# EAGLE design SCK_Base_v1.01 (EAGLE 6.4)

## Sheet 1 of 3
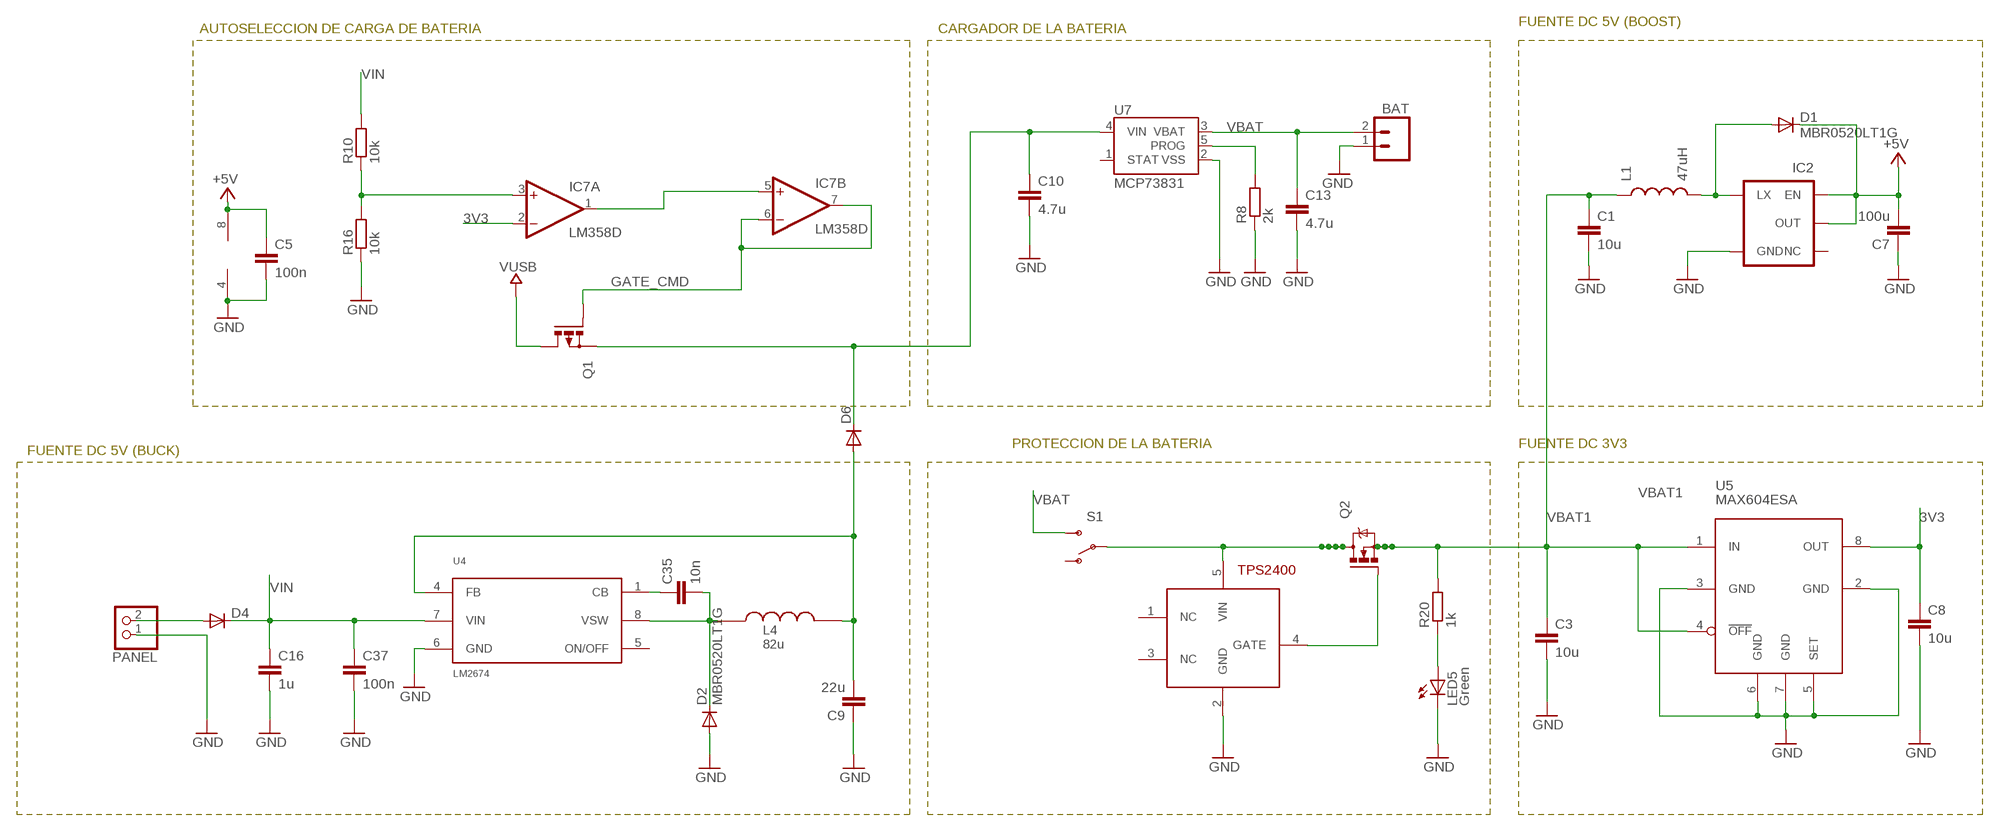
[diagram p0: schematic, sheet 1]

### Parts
BAT  M02-JST-2MM-SMT  [S2B-PH]
C1  10u  C-EUC0805  [C0805]
C3  10u  C-EUC0805  [C0805]
C5  100n  C-EUC0805  [C0805]
C7  100u  C-EUC1206  [C1206]
C8  10u  C-EUC0805  [C0805]
C9  22u  C-EUC1206  [C1206]
C10  4.7u  C-EUC0805  [C0805]
C13  4.7u  C-EUC0805  [C0805]
C16  1u  C-EUC0805  [C0805]
C35  10n  C-EUC0805  [C0805]
C37  100n  C-EUC0805  [C0805]
D1  MBR0520LT1G  DIODE-SOD123  [SOD123]
D2  MBR0520LT1G  DIODE-SOD123  [SOD123]
D4  DIODESMA-ALT  [SMA-DIODE_ALT]
D6  DIODESMA-ALT  [SMA-DIODE_ALT]
IC2  V_REG_NCP1400SOT23-5  [SOT23-5]
IC7  LM358D  [SO08]
L1  47uH  INDUCTORCR54  [CR54]
L4  82u  LSDR1006  [SDR1006]
LED5  Green  LEDCHIP-LED0805  [CHIP-LED0805]
PANEL  PINHD-1X2  [1X02]
Q1  P-MOSFET-SO8  [SO-08]
Q2  N-MOSFET-SO8S  [SO-08]
R8  2k  R-EU_R0805  [R0805]
R10  10k  R-EU_R0805  [R0805]
R16  10k  R-EU_R0805  [R0805]
R20  1k  R-EU_R0805  [R0805]
S1  SWITCH-SPST-SMD-A  [SWITCH-SPST-SMD-A]
U3  TPS2400  [SOT23-5L]
U4  LM2674  [SO8]
U5  MAX604ESA  [SO-08]
U7  MCP73831  [SOT23-5]

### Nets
3V3: C8.1 IC7.2(A:-IN) U5.8(OUT) ; also sheet 3
+5V [usbvcc]: C5.1 C7.2 D1.C IC2.1(EN) IC2.2(OUT) IC7.8(P:V+) ; also sheet 2,3
GATE_CMD: IC7.6(B:-IN) IC7.7(B:OUT) Q1.4(G)
GND: BAT.1 C1.2 C3.2 C5.2 C7.1 C8.2 C9.1 C10.2 C13.2 C16.2 C37.2 D2.A IC2.4(GND) IC7.4(P:V-) LED5.C PANEL.1 R8.1 R16.1 U3.2(GND) U4.6(GND) U5.2(GND) U5.3(GND) U5.5(SET) U5.6(GND) U5.7(GND) U7.2(VSS) ; also sheet 2,3
N$3 [power]: D4.A PANEL.2
N$5: IC7.3(A:+IN) R10.1 R16.2
N$7: IC7.1(A:OUT) IC7.5(B:+IN)
N$10 [usbvcc]: C9.2 D6.A L4.2 U4.4(FB)
N$13: R8.2 U7.5(PROG)
N$19 [usbvcc]: C10.1 D6.C Q1.1(S) Q1.2(S) Q1.3(S) U7.4(VIN)
N$20: LED5.A R20.1
N$30: Q2.4(G) U3.4(GATE)
N$31: D1.A IC2.5(LX) L1.P$2
N$47: C35.1 U4.1(CB)
N$54: C35.2 D2.C L4.1 U4.8(VSW)
VBAT: BAT.2 C13.1 S1.3(S) U7.3(VBAT)
VBAT1: C1.1 C3.1 L1.P$1 Q2.1(S) Q2.2(S) Q2.3(S) R20.2 U5.1(IN) U5.4(!OFF) ; also sheet 2
VIN [power]: C16.1 C37.1 D4.C R10.2 U4.7(VIN) ; also sheet 3
VTPS: Q2.5(D) Q2.6(D) Q2.7(D) Q2.8(D) S1.2(P) U3.5(VIN)
VUSB: Q1.5(D) Q1.6(D) Q1.7(D) Q1.8(D) ; also sheet 2
Unconnected: IC2.3(NC) S1.1(O) U3.1(NC) U3.3(NC) U4.5(ON/OFF) U7.1(STAT)

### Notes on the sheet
- FUENTE DC 5V (BOOST)
- AUTOSELECCION DE CARGA DE BATERIA | CARGADOR DE LA BATERIA
- PROTECCION DE LA BATERIA | FUENTE DC 3V3
- FUENTE DC 5V (BUCK)

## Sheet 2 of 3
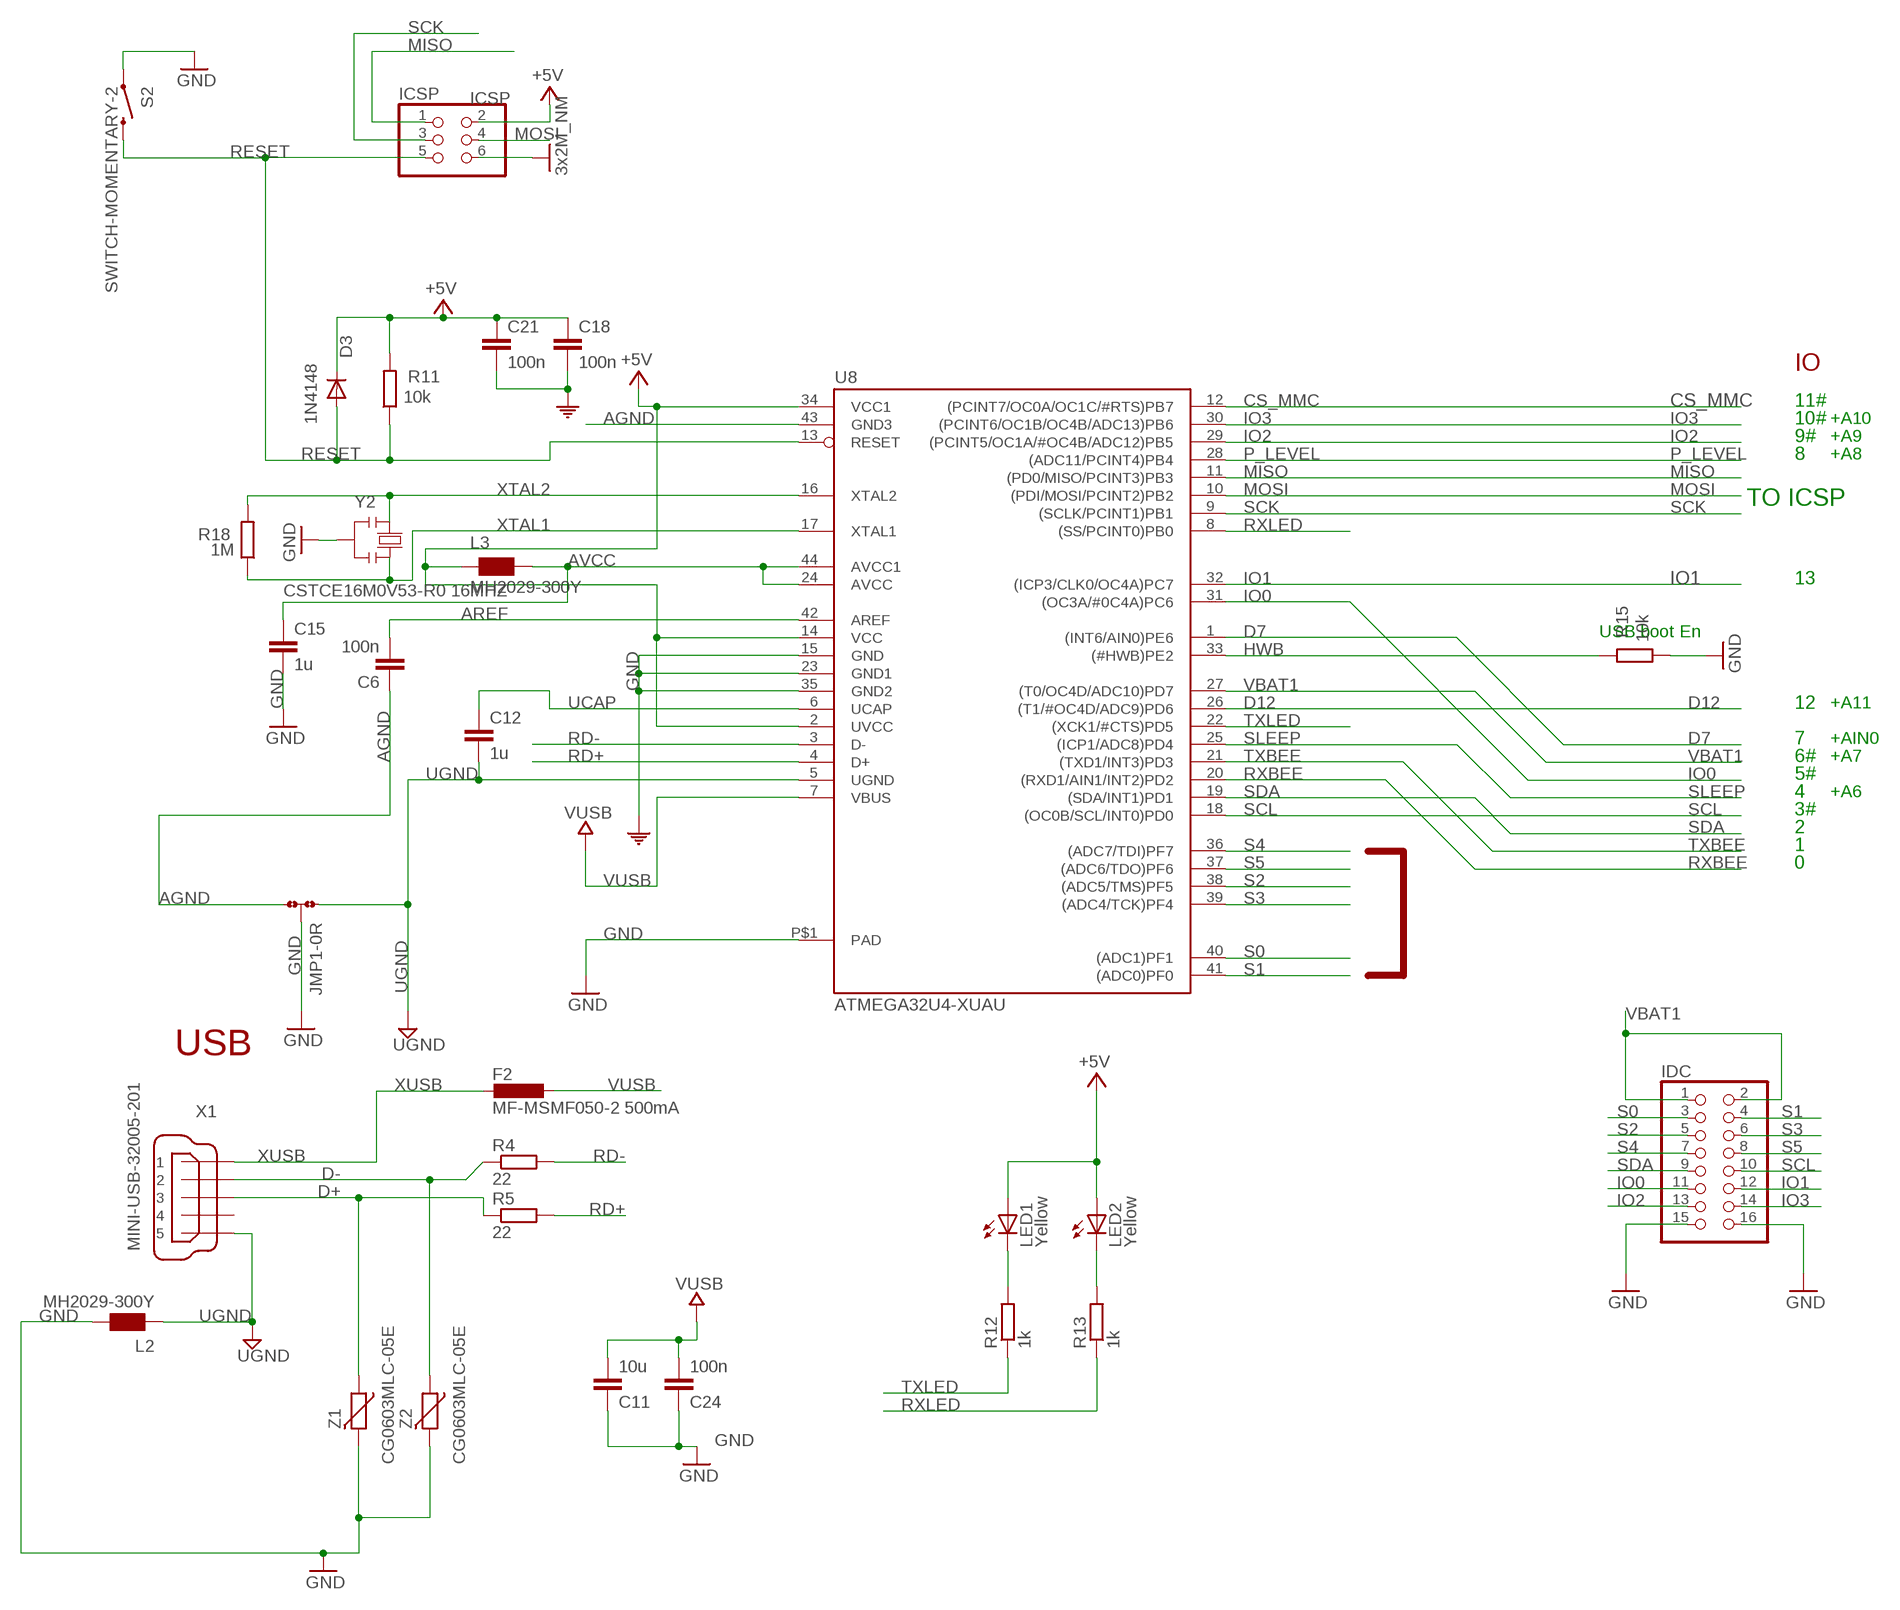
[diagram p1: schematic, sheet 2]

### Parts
C6  100n  C-EUC0805  [C0805]
C11  10u  C-EUC0805  [C0805]
C12  1u  C-EUC0805  [C0805]
C15  1u  C-EUC0805  [C0805]
C18  100n  C-EUC0805  [C0805]
C21  100n  C-EUC0805  [C0805]
C24  100n  C-EUC0805  [C0805]
D3  1N4148  DIODE-SOD123  [SOD123]
F2  MF-MSMF050-2 500mA  L-EUL1812  [L1812]
ICSP  ICSP  PINHD-2X3  [2X03]
IDC  PINHD-2X8  [2X08]
JMP1  0R-JUMPC  [C0R-JMP]
L2  MH2029-300Y  WE-CBF_0805  [0805]
L3  MH2029-300Y  WE-CBF_0805  [0805]
LED1  Yellow  LEDCHIP-LED0805  [CHIP-LED0805]
LED2  Yellow  LEDCHIP-LED0805  [CHIP-LED0805]
R4  22  R-EU_R0805  [R0805]
R5  22  R-EU_R0805  [R0805]
R11  10k  R-EU_R0805  [R0805]
R12  1k  R-EU_R0805  [R0805]
R13  1k  R-EU_R0805  [R0805]
R15  10k  R-EU_R0805  [R0805]
R18  1M  R-EU_R0805  [R0805]
S2  SWITCH-MOMENTARY-2  [TACTILE_SWITCH_TALL]
U8  ATMEGA32U4-XUAU  [TQFP44-PAD]
X1  MINI-USB-32005-201  [32005-201]
Y2  CSTCE16M0V53-R0 16MHZ  RESONATORMU  [RESONATOR]
Z1  CG0603MLC-05E  VARISTORCN0603  [CT/CN0603]
Z2  CG0603MLC-05E  VARISTORCN0603  [CT/CN0603]

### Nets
+5V [usbvcc]: C18.1 C21.1 D3.C ICSP.2 L3.1 LED1.A LED2.A R11.2 U8.2(UVCC) U8.14(VCC) U8.34(VCC1) ; also sheet 1,3
AGND: C6.1 JMP1.3 U8.43(GND3)
AREF [aref]: C6.2 U8.42(AREF)
AVCC: C15.1 L3.2 U8.24(AVCC) U8.44(AVCC1)
CS_MMC: U8.12((PCINT7/OC0A/OC1C/#RTS)PB7) ; also sheet 3
D7: U8.1((INT6/AIN0)PE6)
D12: U8.26((T1/#OC4D/ADC9)PD6)
D+: R5.1 X1.3 Z1.1
D-: R4.1 X1.2 Z2.1
GND: C11.1 C15.2 C18.2 C21.2 C24.1 ICSP.6 IDC.15 IDC.16 JMP1.2 L2.2 R15.1 S2.A2 U8.15(GND) U8.23(GND1) U8.35(GND2) U8.P$1(PAD) Y2.2 Z1.2 Z2.2 ; supply symbol labelled 3x2M_NM, COM ; also sheet 1,3
HWB: R15.2 U8.33((#HWB)PE2)
IO0: IDC.11 U8.31((OC3A/#0C4A)PC6)
IO1: IDC.12 U8.32((ICP3/CLK0/OC4A)PC7)
IO2: IDC.13 U8.29((PCINT5/OC1A/#OC4B/ADC12)PB5)
IO3: IDC.14 U8.30((PCINT6/OC1B/OC4B/ADC13)PB6)
MISO: ICSP.1 U8.11((PD0/MISO/PCINT3)PB3) ; also sheet 3
MOSI: ICSP.4 U8.10((PDI/MOSI/PCINT2)PB2) ; also sheet 3
N$2 [usbvcc]: LED1.C R12.2
N$4 [usbvcc]: LED2.C R13.2
P_LEVEL: U8.28((ADC11/PCINT4)PB4) ; also sheet 3
RD+: R5.2 U8.4(D+)
RD-: R4.2 U8.3(D-)
RESET: D3.A ICSP.5 R11.1 S2.B2 U8.13(RESET) ; also sheet 3
RXBEE: U8.20((RXD1/AIN1/INT2)PD2) ; also sheet 3
RXLED: R13.1 U8.8((SS/PCINT0)PB0)
S0: IDC.3 U8.40((ADC1)PF1)
S1: IDC.4 U8.41((ADC0)PF0)
S2: IDC.5 U8.38((ADC5/TMS)PF5)
S3: IDC.6 U8.39((ADC4/TCK)PF4)
S4: IDC.7 U8.36((ADC7/TDI)PF7)
S5: IDC.8 U8.37((ADC6/TDO)PF6)
SCK: ICSP.3 U8.9((SCLK/PCINT1)PB1) ; also sheet 3
SCL: IDC.10 U8.18((OC0B/SCL/INT0)PD0) ; also sheet 3
SDA: IDC.9 U8.19((SDA/INT1)PD1) ; also sheet 3
SLEEP: U8.25((ICP1/ADC8)PD4) ; also sheet 3
TXBEE: U8.21((TXD1/INT3)PD3) ; also sheet 3
TXLED: R12.1 U8.22((XCK1/#CTS)PD5)
UCAP: C12.1 U8.6(UCAP)
UGND [gnd]: C12.2 JMP1.1 L2.1 U8.5(UGND) X1.5
VBAT1: IDC.1 IDC.2 U8.27((T0/OC4D/ADC10)PD7) ; also sheet 1
VUSB: C11.2 C24.2 F2.1 U8.7(VBUS) ; also sheet 1
XTAL1: R18.1 U8.17(XTAL1) Y2.3
XTAL2: R18.2 U8.16(XTAL2) Y2.1
XUSB [usbvcc]: F2.2 X1.1
Unconnected: X1.4

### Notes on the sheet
- IO
- 11#
- 10# | +A10
- 9# | +A9
- 8 | +A8
- TO ICSP
- 13
- USB boot En
- 12 | +A11
- 7 | +AIN0
- 6# | +A7
- 5#
- 4 | +A6
- 3#
- 2
- 1
- 0
- USB

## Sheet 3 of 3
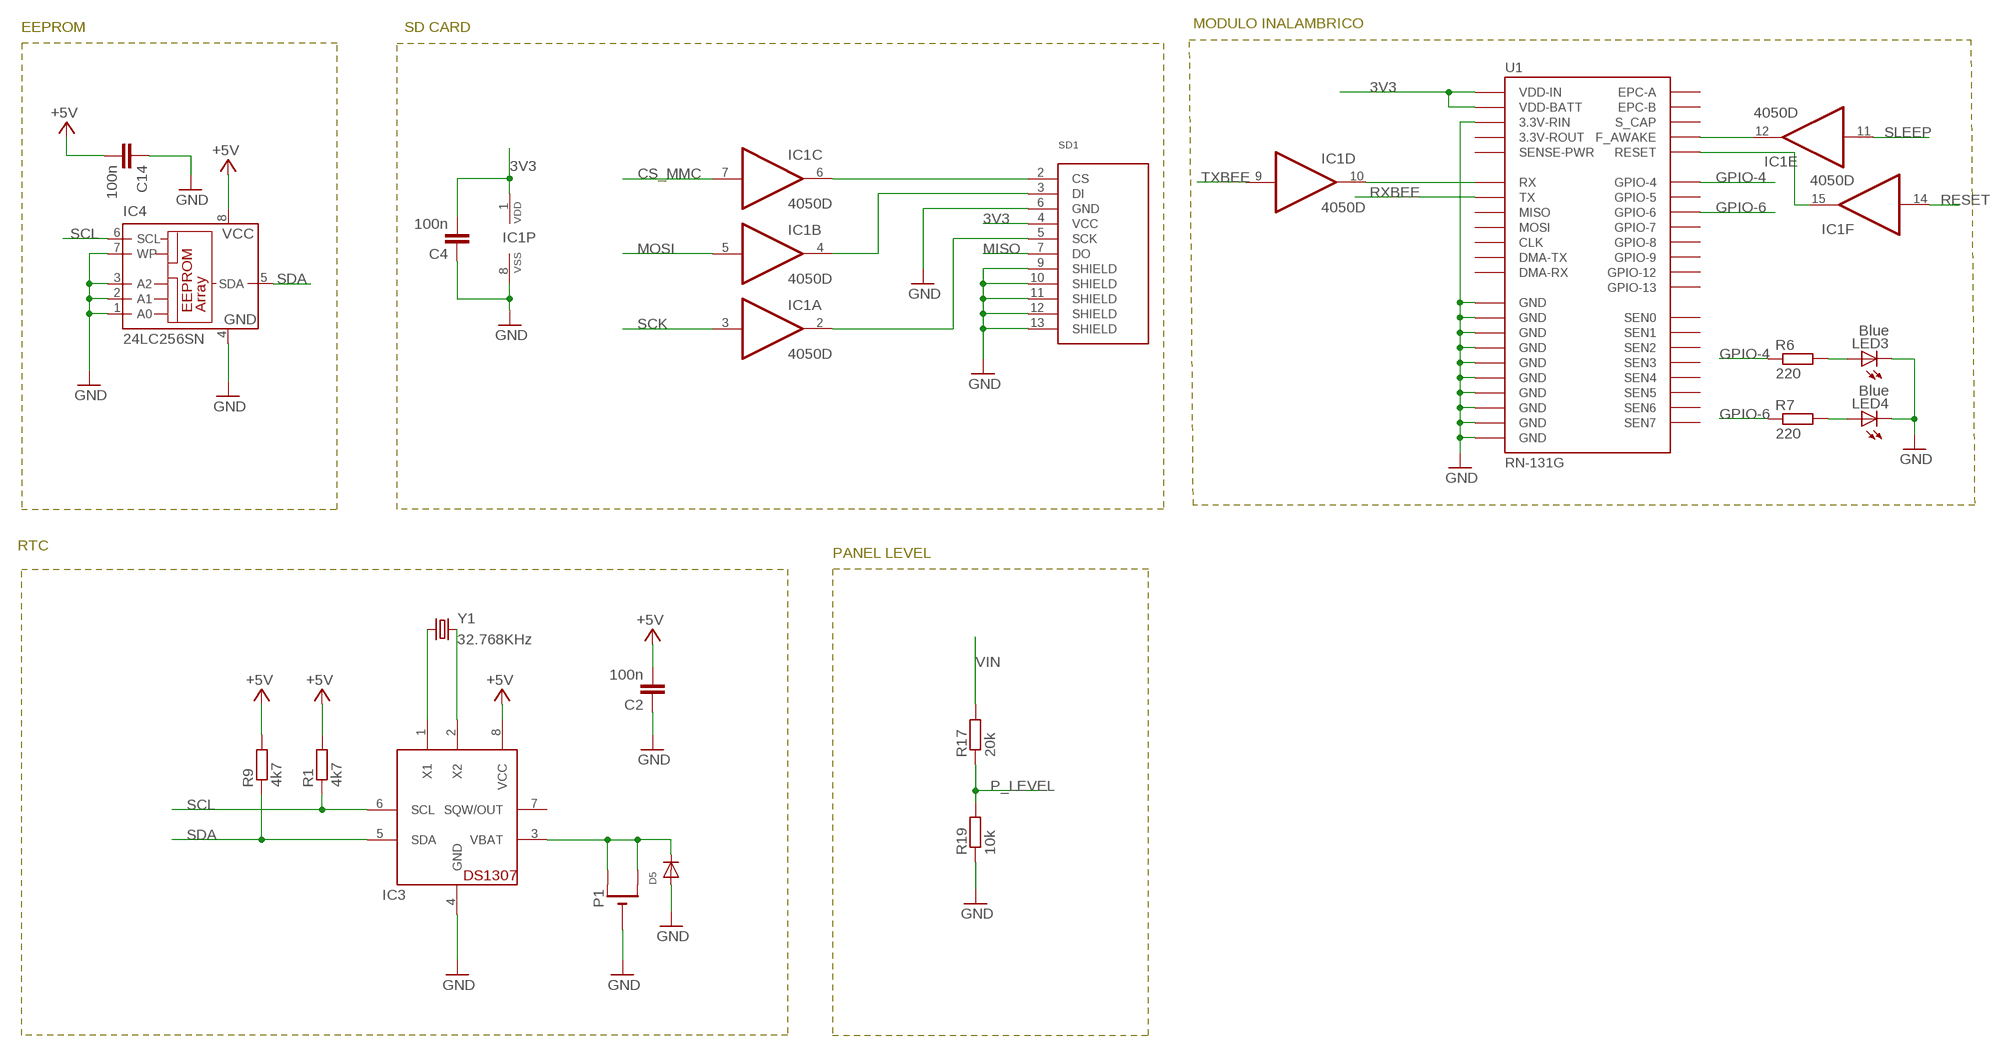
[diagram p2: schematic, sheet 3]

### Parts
C2  100n  C-EUC0805  [C0805]
C4  100n  C-EUC0805  [C0805]
C14  100n  C-EUC0805  [C0805]
D5  DIODESOD-323F  [SOD-323F]
IC1  4050D  [SO16]
IC3  DS1307SOIC  [SO08-SKINNYPADS]
IC4  24LC256SN  [SO-08]
LED3  Blue  LEDCHIP-LED0805  [CHIP-LED0805]
LED4  Blue  LEDCHIP-LED0805  [CHIP-LED0805]
P1  CR1220SMT  [CR1220-SMD]
R1  4k7  R-EU_R0805  [R0805]
R6  220  R-EU_R0805  [R0805]
R7  220  R-EU_R0805  [R0805]
R9  4k7  R-EU_R0805  [R0805]
R17  20k  R-EU_R0805  [R0805]
R19  10k  R-EU_R0805  [R0805]
SD1  SD_CARD_SOCKETDM3CS  [DM3CS]
U1  RN-131G  [RN-131G]
Y1  32.768KHz  CRYSTALABS10  [ABS10]

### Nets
3V3: C4.2 IC1.1(P:VDD) SD1.4(VCC) U1.P$20(VDD-BATT) U1.P$21(VDD-IN) ; also sheet 1
+5V [usbvcc]: C2.2 C14.2 IC3.8(VCC) IC4.8(VCC) R1.2 R9.2 ; also sheet 1,2
CS_MMC: IC1.7(C:I) ; also sheet 2
GND: C2.1 C4.1 C14.1 D5.A IC1.8(P:VSS) IC3.4(GND) IC4.1(A0) IC4.2(A1) IC4.3(A2) IC4.4(GND) IC4.7(WP) LED3.C LED4.C P1.- R19.1 SD1.6(GND) SD1.9(SHIELD) SD1.10(SHIELD) SD1.11(SHIELD) SD1.12(SHIELD) SD1.13(SHIELD) U1.P$18(3.3V-RIN) U1.P$19(GND) U1.P$36(GND) U1.P$37(GND) U1.P$38(GND) U1.P$39(GND) U1.P$40(GND) U1.P$41(GND) U1.P$42(GND) U1.P$43(GND) U1.P$44(GND) ; also sheet 1,2
GPIO-4: R6.1 U1.P$29(GPIO-4)
GPIO-6: R7.1 U1.P$27(GPIO-6)
MISO: SD1.7(DO) ; also sheet 2
MOSI: IC1.5(B:I) ; also sheet 2
N$1: IC1.10(D:O) U1.P$12(RX)
N$6: LED4.A R7.2
N$8: LED3.A R6.2
N$9: IC1.6(C:O) SD1.2(CS)
N$11: IC1.2(A:O) SD1.5(SCK)
N$12: IC1.4(B:O) SD1.3(DI)
N$14: IC1.12(E:O) U1.P$9(F_AWAKE)
N$15: IC1.15(F:O) U1.P$5(RESET)
N$16: IC3.1(X1) Y1.1
N$17: IC3.2(X2) Y1.2
N$18: D5.C IC3.3(VBAT) P1.+$1(+) P1.+$2(+1)
P_LEVEL: R17.1 R19.2 ; also sheet 2
RESET: IC1.14(F:I) ; also sheet 2
RXBEE: U1.P$13(TX) ; also sheet 2
SCK: IC1.3(A:I) ; also sheet 2
SCL: IC3.6(SCL) IC4.6(SCL) R1.1 ; also sheet 2
SDA: IC3.5(SDA) IC4.5(SDA) R9.1 ; also sheet 2
SLEEP: IC1.11(E:I) ; also sheet 2
TXBEE: IC1.9(D:I) ; also sheet 2
VIN [power]: R17.2 ; also sheet 1
Unconnected: IC3.7(SQW/OUT) U1.P$1(SEN6) U1.P$2(SEN4) U1.P$3(SEN5) U1.P$4(SEN7) U1.P$6(EPC-A) U1.P$7(EPC-B) U1.P$8(S_CAP) U1.P$10(GPIO-13) U1.P$11(GPIO-12) U1.P$14(MOSI) U1.P$15(CLK) U1.P$16(MISO) U1.P$17(3.3V-ROUT) U1.P$22(DMA-TX) U1.P$23(DMA-RX) U1.P$24(GPIO-9) U1.P$25(GPIO-8) U1.P$26(GPIO-7) U1.P$28(GPIO-5) U1.P$30(SEN1) U1.P$31(SEN2) U1.P$32(SEN3) U1.P$33(SENSE-PWR) U1.P$34(SEN0)

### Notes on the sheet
- EEPROM | SD CARD | MODULO INALAMBRICO
- RTC
- PANEL LEVEL

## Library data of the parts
BAT = SparkFun:M02: Header 2
C1-C5 C7-C10 C13 C14 C16 C35 C37 = rcl:C-EU: CAPACITOR, European symbol
C6 C11 C12 C15 C18 C21 C24 = SmartPrj:C-EU: CAPACITOR, European symbol
D1-D3 = diode:DIODE-: DIODE
D4 D6 = SparkFun-DiscreteSemi:DIODE: Diode
D5 = adafruit:DIODE: Diode
F2 = rcl:L-EU: INDUCTOR, European symbol
IC1 = 40xx:4050: Hex non-inverting BUFFER
IC2 = SparkFunEagle-3-30-09:V_REG_NCP1400: Switching step-up voltage regulator NCP1400 switiching regulator takes single cell AA and outputs 100mA at 3.3V or 5V with minimal number of external components.
IC3 = adafruit:DS1307: DS1307 Real time clock (RTC) with battery backup ability. Talk to it via i2c
IC4 = microchip:24*: Serial EEPROM I2C; MF: MICROCHIP; MPN: 24LC256-I/SN; OC_FARNELL: 9757996; OC_NEWARK: 27C9144
IC7 = linear:LM358: OP AMP also LM158; LM258; LM2904 Source: http://cache.national.com/ds/LM/LM158.pdf
ICSP = SmartPrj:PINHD-2X3: PIN HEADER
IDC = pinhead:PINHD-2X8: PIN HEADER
JMP1 = jump-0r-smd:0R-JUMP: SMD 0R 0805 Jumper
L1 = SparkFunEagle-3-30-09:INDUCTOR: Inductors
L2 L3 = wuerth-elektronik:WE-CBF: SMD EMI Suppression Ferrite Beads
L4 = Hangar:L
LED1-LED5 = led:LED: LED
P1 = adafruit:CR1220: CR1216/CR1220/CR1225 12mm 3V lithium coin cell Great for battery packup. Both SMT and THM holders. Note the THM package has the ground pads on both sides of the PCB so that the masks are the same - this reduces the cost
PANEL = pinhead:PINHD-1X2: PIN HEADER
Q1 = transistor-power:P-MOSFET-SO8: P-Channel MOSFET Example: FDS4435A; P-Channel Logic Level PowerTrench® MOSFET FDS4465; P-Channel 1.8V Specified PowerTrench® MOSFET Source: www.fairchildsemi.com
Q2 = transistor-power:N-MOSFET-SO8: N-Channel MOSFET Example: FDS7760A; N-Channel Logic Level PowerTrench® MOSFET FDS2572; N-Channel UltraFET® Trench MOSFET Source: www.fairchildsemi.com
R1 R4-R10 R12 R13 R16 R17 R19 R20 = rcl:R-EU_: RESISTOR, European symbol
R11 R15 R18 = SmartPrj:R-EU_: RESISTOR, European symbol
S1 = SparkFun 13-1-2012:SWITCH-SPST: SPST Switch Simple slide switch. Spark Fun Electronics SKU : COM-00102
S2 = SparkFun 13-1-2012:SWITCH-MOMENTARY-2
SD1 = Hangar:SD_CARD_SOCKET: SD/MMC Socket Media socket for SD and MMC cards. Push-push type. Model MOLEX 503182-0853
U1 = SparkFun:RN-131G: Roving Netowrks WiFLy GSX Module
U3 = texas-msp:TPS2400
U4 = Hangar:LM2674
U5 = Hangar:MAX604
U7 = SparkFun-PowerIC:MCP73831: Miniature single cell, fully integrated Li-Ion, Li-polymer charge management controller http://ww1.microchip.com/downloads/en/DeviceDoc/21984a.pdf
U8 = SmartPrj:ATMEGA32U4-XU
X1 = con-cypressindustries:MINI-USB-: MINI USB-B Conector Source: www.cypressindustries.com; OC_FARNELL: unknown; OC_NEWARK: unknown
Y1 = Hangar:CRYSTAL: CRYSTAL
Y2 = SmartPrj:RESONATOR
Z1 Z2 = varistor:VARISTOR: VARISTOR

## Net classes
1 power: width 0.254 mm, drill 0.6 mm, clearance 0.203 mm
2 gnd: width 0.254 mm, drill 0.6 mm, clearance 0.203 mm
3 usbvcc: width 0.254 mm, drill 0.6 mm, clearance 0.203 mm
4 aref: width 0.254 mm, drill 0.6 mm, clearance 0.203 mm

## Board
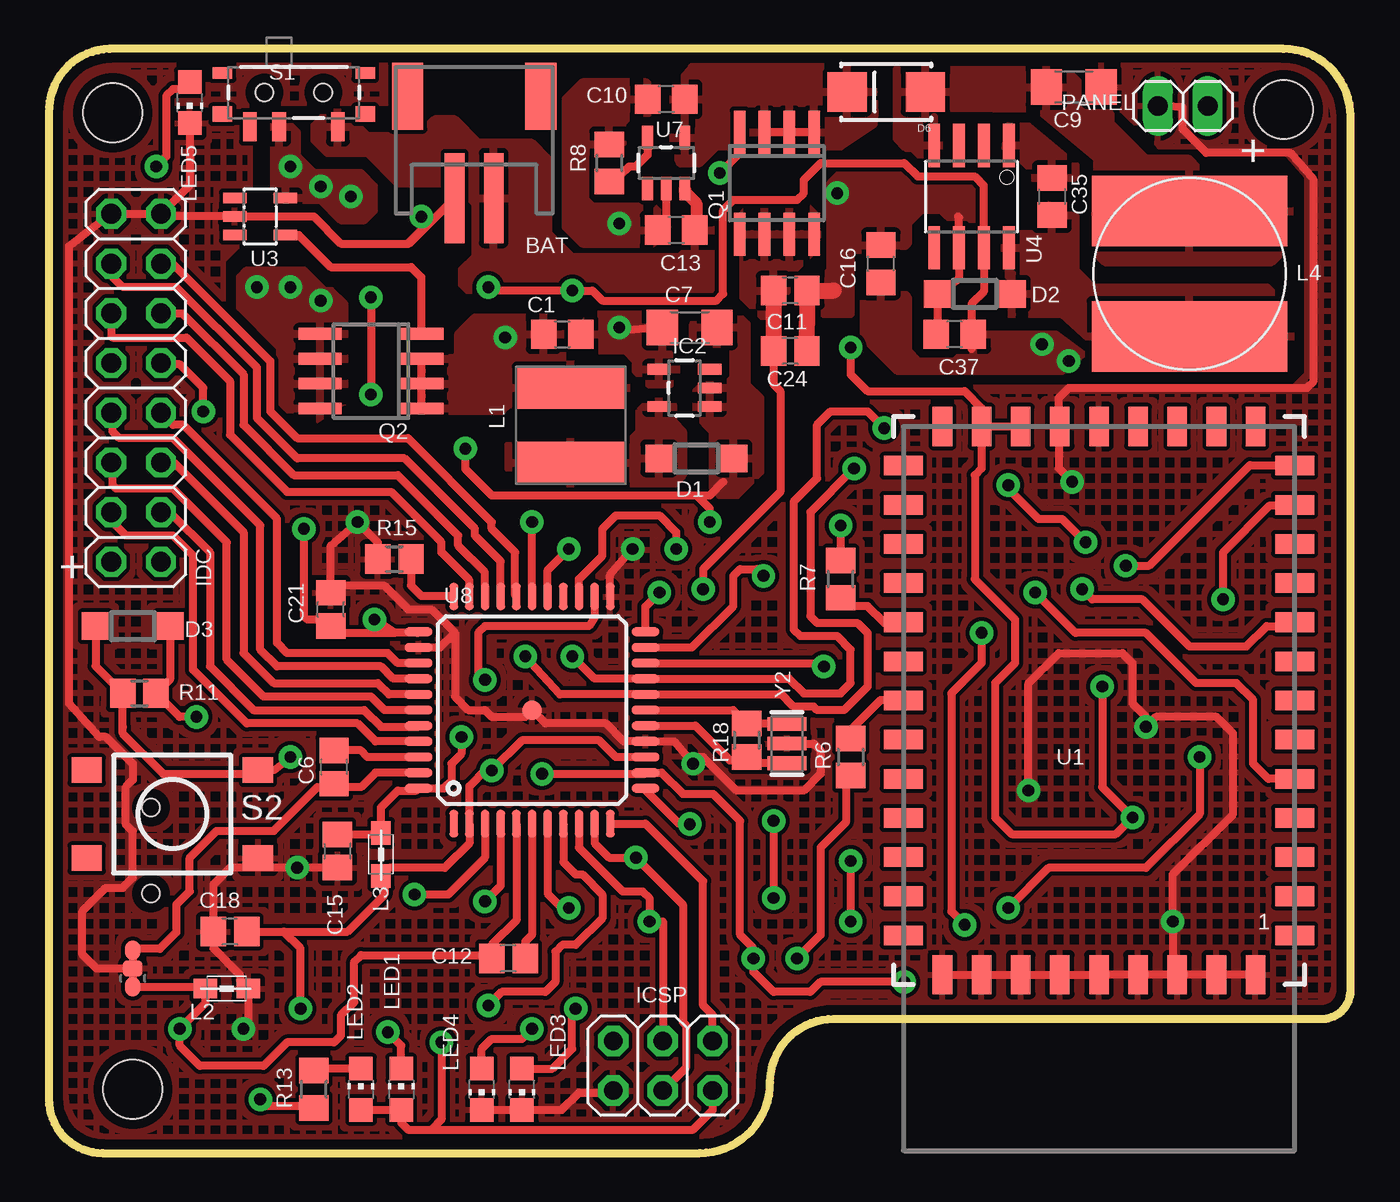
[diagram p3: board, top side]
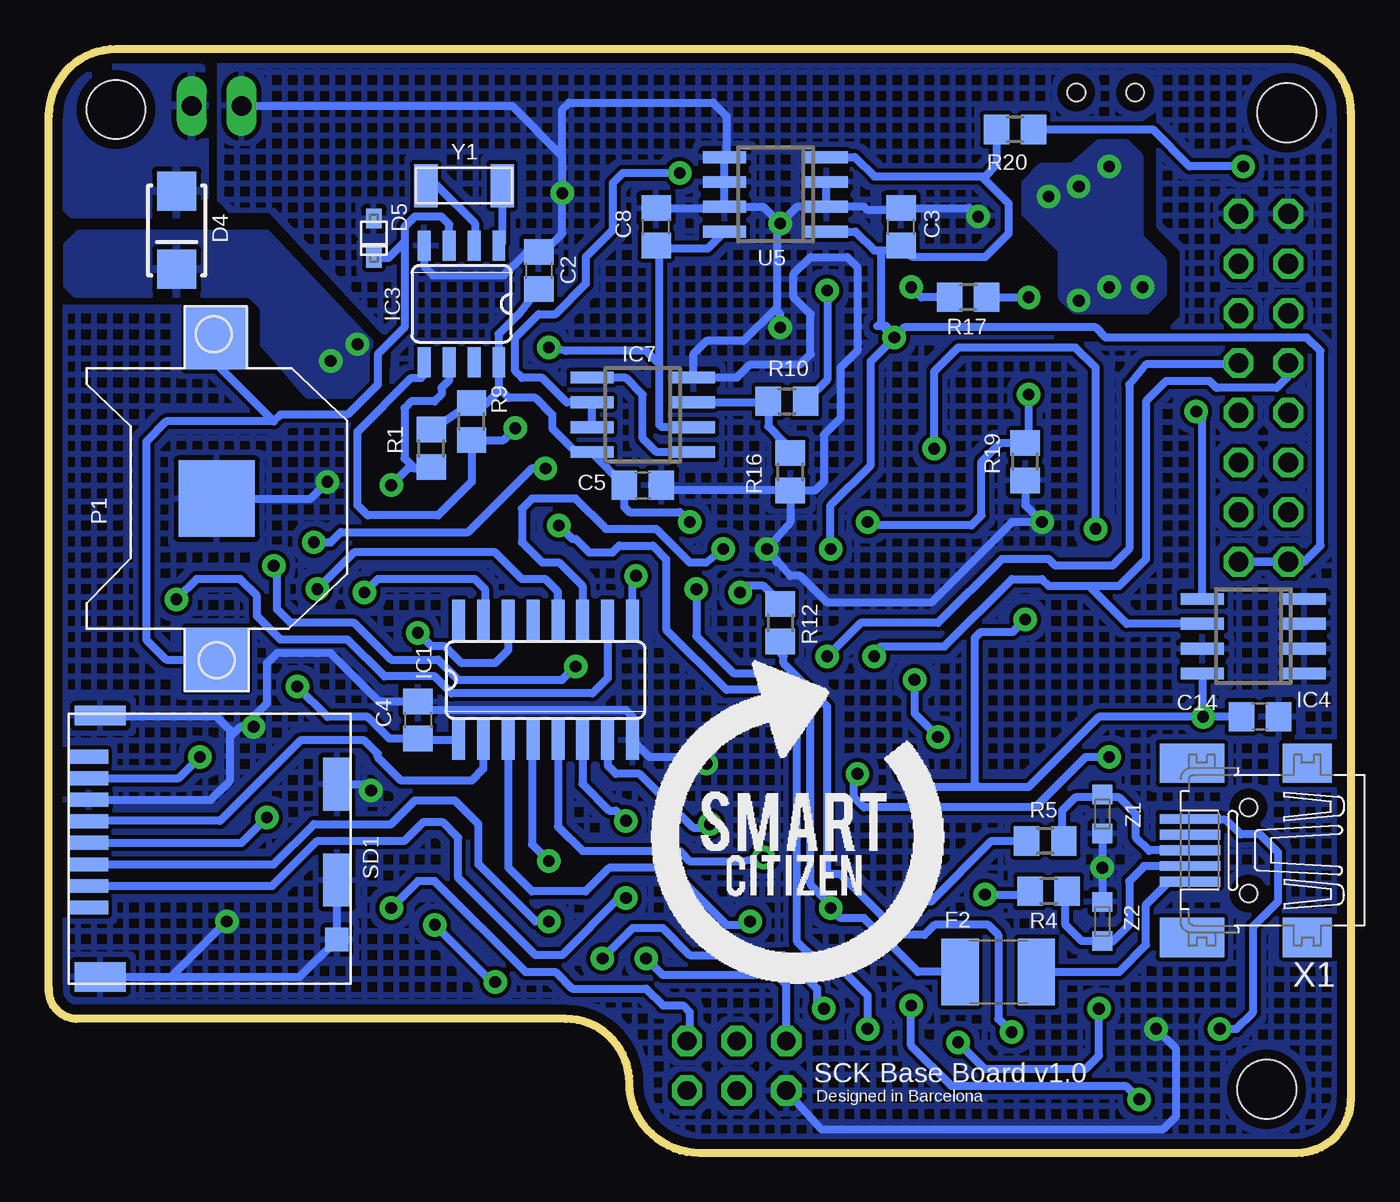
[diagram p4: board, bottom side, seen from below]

Size 66.52 x 56.41 mm. Coordinates in mm from the lower left corner, seen from the top.
Outline: 2.74,0 33.26,0 arc90 36.86,3.6 arc-90 40.12,6.86 65.15,6.86 arc90 66.52,8.4 66.52,52.98 arc90 63.09,56.41 3.09,56.41 arc90 0,53.15 0,2.74 arc90 2.74,0
Copper layers (1*16): Top 0.035mm / dielectric 1.5mm / Bottom 0.035mm
Design rules "default": minimum track width 6mil, minimum drill 0.6mm, track to track 8mil, track to pad 8mil, pad to pad 8mil, via to via 8mil, smd to smd 8mil, copper to edge 20mil, drill to drill 1mm, minimum pad ring 10mil, minimum via ring 0.3mm, stop-mask expansion 4mil, vias tented up to drill 0mil, thermal gap 10mil
Holes 3 mm at 3.26,53.15 4.29,3.26 63.09,53.32

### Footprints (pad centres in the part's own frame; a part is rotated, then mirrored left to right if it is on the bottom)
S2B-PH = smd 1 x 4.6: 1 -1,-3.7; 2 1,-3.7 | smd 1.6 x 3.4: NC1 -3.4,1.5; NC2 3.4,1.5
C0805 = smd 1.3 x 1.5: 1 -0.95,0; 2 0.95,0
C0805' = smd 1.3 x 1.5: 1 -0.85,0; 2 0.85,0
C1206 = smd 1.6 x 1.8: 1 -1.4,0; 2 1.4,0
SOD123 = smd 1.4 x 1.4: A 1.9,0; C -1.9,0
SMA-DIODE_ALT = smd 2 x 2: A -2,0; C 2,0
SOD-323F = smd 1 x 0.8: A -1,0; C 1,0
L1812 = smd 1.9 x 3.4: 1 -1.95,0; 2 1.95,0
SO16 = smd 0.66 x 2.032: 1 -4.445,-3.073; 2 -3.175,-3.073; 3 -1.905,-3.073; 4 -0.635,-3.073; 5 0.635,-3.073; 6 1.905,-3.073; 7 3.175,-3.073; 8 4.445,-3.073; 9 4.445,3.073; 10 3.175,3.073; 11 1.905,3.073; 12 0.635,3.073; 13 -0.635,3.073; 14 -1.905,3.073; 15 -3.175,3.073; 16 -4.445,3.073
SOT23-5 = smd 0.55 x 1.2: 1 -0.95,-1.3; 2 0,-1.3; 3 0.95,-1.3; 4 0.95,1.3; 5 -0.95,1.3
SO08-SKINNYPADS = smd 0.66 x 1.524: 1 -1.905,-2.973; 2 -0.635,-2.973; 3 0.635,-2.973; 4 1.905,-2.973; 5 1.905,2.973; 6 0.635,2.973; 7 -0.635,2.973; 8 -1.905,2.973
SO-08 = smd 0.6 x 2.2: 1 -1.905,-2.6; 2 -0.635,-2.6; 3 0.635,-2.6; 4 1.905,-2.6; 5 1.905,2.6; 6 0.635,2.6; 7 -0.635,2.6; 8 -1.905,2.6
SO08 = smd 0.6 x 2.2: 1 -1.905,-2.6; 2 -0.635,-2.6; 3 0.635,-2.6; 4 1.905,-2.6; 5 1.905,2.6; 6 0.635,2.6; 7 -0.635,2.6; 8 -1.905,2.6
2X03 = drill 0.95 pad 1.55 octagon: 1 -2.54,-1.27; 2 -2.54,1.27; 3 0,-1.27; 4 0,1.27; 5 2.54,-1.27; 6 2.54,1.27
2X08 = drill 1.016 octagon: 1 -8.89,-1.27; 2 -8.89,1.27; 3 -6.35,-1.27; 4 -6.35,1.27; 5 -3.81,-1.27; 6 -3.81,1.27; 7 -1.27,-1.27; 8 -1.27,1.27; 9 1.27,-1.27; 10 1.27,1.27; 11 3.81,-1.27; 12 3.81,1.27; 13 6.35,-1.27; 14 6.35,1.27; 15 8.89,-1.27; 16 8.89,1.27
C0R-JMP = smd 0.8 x 1: 1 0,0.938; 3 0,-0.938 | smd 1 x 0.8: 2 0,0
CR54 = smd 5.5 x 2.15: P$1 0,1.92; P$2 0,-1.92
0805 = smd 1.2 x 1: 1 -1.1,0; 2 1.1,0
SDR1006 = smd 10 x 3.6: 1 0,3.2; 2 0,-3.2
CHIP-LED0805 = smd 1.2 x 1.2: A 0,-1.05; C 0,1.05
CR1220-SMD = smd 3.2 x 3.2: +$1 -8.2,0; +$2 8.2,0 | smd 3.9 x 3.9: - 0,0
1X02 = drill 1.016 long: 1 -1.27,0; 2 1.27,0
R0805 = smd 1.3 x 1.5: 1 -0.95,0; 2 0.95,0
R0805' = smd 1.3 x 1.5: 1 -0.85,0; 2 0.85,0
SWITCH-SPST-SMD-A = smd 0.7 x 1.5: 1 -2.25,-1.75; 2 -0.75,-1.75; 3 2.25,-1.75 | smd 1 x 0.6: GND1 -3.65,1; GND3 3.65,1 | smd 1 x 0.8: GND2 -3.65,-1.1; GND4 3.65,-1.1 | hole 0.9: -1.5,0; 1.5,0
TACTILE_SWITCH_TALL = smd 1.55 x 1.3: A1 -4.375,-2.25; A2 4.375,-2.25; B1 -4.375,2.25; B2 4.375,2.25
DM3CS = smd 0.7 x 2: 1 2.54,-5.35; 2 1.44,-5.35; 3 0.34,-5.35; 4 -0.76,-5.35; 5 -1.86,-5.35; 6 -2.96,-5.35; 7 -4.06,-5.35; 8 -5.16,-5.35 | smd 1 x 2.6: 9 -7.26,-4.75 | smd 2.7 x 1.4: 10 -3.76,7.35; 11 1.14,7.35 | smd 1.2 x 1.2: 12 4.19,7.35 | smd 1.5 x 2.6: 13 6.09,-4.75
RN-131G = smd 2 x 1: P$1 -10,11; P$2 -10,9; P$3 -10,7; P$4 -10,5; P$5 -10,3; P$6 -10,1; P$7 -10,-1; P$8 -10,-3; P$9 -10,-5; P$10 -10,-7; P$11 -10,-9; P$12 -10,-11; P$13 -10,-13; P$23 10,-13; P$24 10,-11; P$25 10,-9; P$26 10,-7; P$27 10,-5; P$28 10,-3; P$29 10,-1; P$30 10,1; P$31 10,3; P$32 10,5; P$33 10,7; P$34 10,9; P$35 10,11 | smd 1 x 2: P$14 -8,-15; P$15 -6,-15; P$16 -4,-15; P$17 -2,-15; P$18 0,-15; P$19 2,-15; P$20 4,-15; P$21 6,-15; P$22 8,-15; P$36 8,13; P$37 6,13; P$38 4,13; P$39 2,13; P$40 0,13; P$41 -2,13; P$42 -4,13; P$43 -6,13; P$44 -8,13
SOT23-5L = smd 0.55 x 1.2: 1 -0.95,-1.3; 2 0,-1.3; 3 0.95,-1.3; 4 0.95,1.3; 5 -0.95,1.3
SO8 = smd 0.61 x 2.21: 1 -1.905,-2.616; 2 -0.635,-2.616; 3 0.635,-2.616; 4 1.905,-2.616; 5 1.905,2.616; 6 0.635,2.616; 7 -0.635,2.616; 8 -1.905,2.616
TQFP44-PAD = smd 1.4 x 0.45: 1 -5.8,4; 2 -5.8,3.2; 3 -5.8,2.4; 4 -5.8,1.6; 5 -5.8,0.8; 6 -5.8,0; 7 -5.8,-0.8; 8 -5.8,-1.6; 9 -5.8,-2.4; 10 -5.8,-3.2; 11 -5.8,-4; 23 5.8,-4; 24 5.8,-3.2; 25 5.8,-2.4; 26 5.8,-1.6; 27 5.8,-0.8; 28 5.8,0; 29 5.8,0.8; 30 5.8,1.6; 31 5.8,2.4; 32 5.8,3.2; 33 5.8,4 | smd 0.45 x 1.4: 12 -4,-5.8; 13 -3.2,-5.8; 14 -2.4,-5.8; 15 -1.6,-5.8; 16 -0.8,-5.8; 17 0,-5.8; 18 0.8,-5.8; 19 1.6,-5.8; 20 2.4,-5.8; 21 3.2,-5.8; 22 4,-5.8; 34 4,5.8; 35 3.2,5.8; 36 2.4,5.8; 37 1.6,5.8; 38 0.8,5.8; 39 0,5.8; 40 -0.8,5.8; 41 -1.6,5.8; 42 -2.4,5.8; 43 -3.2,5.8; 44 -4,5.8 | smd 1 x 1: P$1 0,0
32005-201 = smd 3.1 x 0.5: 1 3,1.6; 2 3,0.8; 3 3,0; 4 3,-0.8; 5 3,-1.6 | smd 2.5 x 2: M1 -3,-4.45; M2 -3,4.45 | smd 3.3 x 2: M3 2.9,4.45; M4 2.9,-4.45 | hole 0.9: 0,2.2; 0,-2.2
ABS10 = smd 1.2 x 2.2: 1 -1.9,-0.05; 2 2,-0.05
RESONATOR = smd 0.7 x 2: 1 -1,0; 2 0,0; 3 1,0
CT/CN0603 = smd 1 x 1: 1 -1,0; 2 1,0

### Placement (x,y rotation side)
BAT  21.73,52.49 0 top
C1  26.23,41.83 0 top
C2  41.49,45.09 270 bottom
C3  22.97,47.32 90 bottom
C4  47.66,22.12 270 bottom
C5  36.18,34.12 0 bottom
C6  100n  [C0805']  14.57,19.72 90 top
C7  32.75,42.18 0 top
C8  35.49,47.32 90 bottom
C9  52.38,54.46 180 top
C10  31.55,53.84 180 top
C11  10u  [C0805']  37.89,44.06 180 top
C12  1u  [C0805']  23.49,9.94 180 top
C13  32.06,47.15 180 top
C14  4.63,22.29 180 bottom
C15  1u  [C0805']  14.74,15.43 270 top
C16  42.52,45.43 90 top
C18  100n  [C0805']  9.26,11.32 180 top
C21  100n  [C0805']  14.4,27.77 90 top
C24  100n  [C0805']  37.89,40.98 180 top
C35  51.26,48.86 270 top
C37  46.29,41.83 180 top
D1  33.09,35.49 180 top
D2  47.32,43.89 180 top
D3  4.29,26.92 180 top
D4  60,47.14 270 bottom
D5  49.92,46.74 270 bottom
D6  42.79,54.21 180 top
F2  18,9.26 0 bottom
IC1  41.15,24.17 0 bottom
IC2  32.48,39.09 90 top
IC3  45.43,43.38 180 bottom
IC4  4.97,26.4 90 bottom
IC7  36.18,37.72 90 bottom
ICSP  31.38,4.46 180 top
IDC  4.46,39.09 90 top
JMP1  4.29,9.43 180 top
L1  26.67,37.18 0 top
L2  9.09,8.4 0 top
L3  16.97,15.26 90 top
L4  58.29,44.92 180 top
LED1  18,3.26 0 top
LED2  15.94,3.26 0 top
LED3  24.17,3.26 180 top
LED4  22.12,3.26 180 top
LED5  7.2,53.66 180 top
P1  57.95,33.43 90 bottom
PANEL  57.95,53.49 0 top
Q1  37.2,49.55 180 top
Q2  16.46,39.95 90 top
R1  46.98,36 90 bottom
R4  15.43,13.37 180 bottom
R5  15.6,15.94 180 bottom
R6  40.98,20.23 270 top
R7  40.46,29.32 90 top
R8  28.63,50.58 270 top
R9  44.92,37.38 90 bottom
R10  28.8,38.4 0 bottom
R11  10k  [R0805']  4.63,23.49 0 top
R12  29.15,27.09 270 bottom
R13  13.54,3.26 90 top
R15  10k  [R0805']  17.66,30.35 0 top
R16  28.63,34.8 90 bottom
R17  19.55,43.72 180 bottom
R18  1M  [R0805']  35.66,21.09 270 top
R19  16.63,35.32 90 bottom
R20  17.14,52.29 180 bottom
S1  12.52,54.18 0 top
S2  6.31,17.32 0 top
SD1  59.15,15.09 270 bottom
U1  53.66,22.12 180 top
U3  10.79,47.85 270 top
U4  47.15,48.86 180 top
U5  29.39,48.97 90 bottom
U7  31.55,50.58 0 top
U8  24.69,22.63 90 top
X1  5.21,15.46 180 bottom
Y1  45.26,49.38 180 bottom
Y2  37.72,20.92 90 top
Z1  12.69,17.32 270 bottom
Z2  12.69,11.83 90 bottom

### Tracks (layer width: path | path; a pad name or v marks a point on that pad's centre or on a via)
3V3  (via drill 0.6)
  Top 0.406: v53.84,23.83 53.84,18.69 v55.38,17.15 54.52,16.29 49.21,16.29 48.35,17.15 48.35,24 49.38,25.03 49.38,27.26 47.32,29.32 47.32,34.63 47.66,34.98 U1.P$21 | v40.98,41.15 40.98,39.78 41.83,38.92 46.81,38.92 47.66,38.06 U1.P$21 | U1.P$21 U1.P$20
  Bottom 0.406: 53.32,23.32 v53.84,23.83 52.29,22.29 50.23,22.29 49.11,21.17 C4.2 47.6,21.1 IC1.1 | v55.38,17.15 56.68,15.85 SD1.4 | IC7.2 35.2,37.08 35.32,37.21 35.32,40.29 | 35.32,40.29 35.32,43.14 35.33,43.15 35.33,46.21 | 35.33,46.21 C8.1 | 35.33,46.21 32.85,46.21 U5.8 | 35.32,40.29 36,40.98 40.12,40.98 v40.98,41.15
+5V  (via drill 0.6)
  Top 0.406: 17.66,26.58 14.74,26.58 C21.1 14.07,27.26 13.2,27.26 13.03,27.43 v13.03,31.89 | U8.34 18.83,26.58 17.66,26.58 | 17.66,26.58 v16.63,27.26 | v7.54,22.29 6.68,22.29 R11.2 6.19,24.2 D3.C | ICSP.2 33.92,2.2 32.92,1.2 19.55,1.2 | LED2.A LED1.A 18,1.54 18.35,1.2 19.55,1.2 | U8.14 28.97,20.23 28.12,21.09 24.17,21.09 v22.63,19.55 22.29,19.55 21.49,18.75 U8.2 21.49,15.83 20.23,14.57 17.39,14.57 L3.1 17.15,13.99 17.15,13.2 15.26,11.32 12,11.32 | v20.06,5.66 20.06,1.71 19.55,1.2 | C18.1 12,11.32 | v12.86,7.37 12.86,10.46 12,11.32 | 33.09,33.6 22.63,33.6 21.28,34.96 v21.28,35.99 | 33.09,33.6 33.78,33.6 34.46,34.29 | v33.78,32.23 33.78,32.92 33.09,33.6
  Bottom 0.406: R1.2 R9.2 44.83,38.23 44.23,38.23 43.55,38.92 43.55,39.09 | 43.49,40.4 IC3.8 43.55,40.42 | 43.55,40.42 43.55,39.09 | 43.55,39.09 43.03,38.58 41.66,38.58 40.81,37.72 40.81,37.03 39.61,35.83 38.8,35.83 IC7.8 38.78,35.77 C5.1 37.13,33.01 36.86,32.75 34.29,32.75 v33.78,32.23 | C2.2 42.44,42.94 43.55,41.83 43.55,40.42 | v13.03,31.89 13.03,40.12 14.06,41.15 20.06,41.15 21.28,39.93 v21.28,35.99 | v20.06,5.66 18.69,4.29 13.54,4.29 12.86,4.97 v12.86,7.37 | v7.54,22.29 12.86,22.29 16.46,18.69 19.03,18.69 | 19.03,18.69 21.77,18.69 v22.63,19.55 | 19.03,18.69 19.2,18.86 19.2,26.32 U8.34 17.26,26.63 v16.63,27.26 | C14.2 v7.54,22.29 | IC4.8 7.57,22.32 v7.54,22.29
  pour Top: 32.92,41.66 32.92,42.35 33.43,42.86 35.15,42.86 35.66,42.35 35.66,39.26 36.35,38.58 36.35,34.8 35.15,33.6 34.29,33.6 33.95,33.95 33.95,36.86 33.09,37.72 33.09,38.92 33.43,39.26 34.63,39.26 34.98,39.6 34.98,40.98 34.63,41.32 33.26,41.32
AGND
  Top 0.406: U8.43 16.69,19.43 15.94,18.69 14.75,18.69 C6.1 14.39,18.69 13.72,18.69 11.49,16.46 8.57,16.46 7.2,15.09 7.2,13.37 6.52,12.69 6.52,11.27 5.67,10.43 4.34,10.43 JMP1.3
AREF
  Top 0.406: U8.42 16.29,20.23 15.94,20.57 14.58,20.57 C6.2
AVCC  (via drill 0.6)
  Top 0.406: C15.1 16.97,16.28 L3.2 16.97,17.66 17.83,18.52 18.77,18.52 U8.44 20.17,18.63 20.57,19.03 20.57,19.89 21.09,20.4 v21.09,21.26 | U8.24 27.89,27.37 27.6,26.92 22.29,26.92 21.95,26.58 21.95,24.52 v22.29,24.17
  Bottom 0.406: v22.29,24.17 22.29,22.46 v21.09,21.26
CS_MMC  (via drill 0.6)
  Top 0.406: U8.12 30.49,18.55 32.23,16.8 v32.75,16.8
  Bottom 0.406: IC1.7 37.97,19.8 37.55,19.37 36.35,19.37 33.6,16.63 32.92,16.63 v32.75,16.8
D+
  Bottom 0.406: 14.62,15.97 R5.1 14.74,16.04 14.74,17.49 14.06,18.17 12.66,18.17 | 12.66,18.17 11.83,18.17 10.97,17.32 10.97,16.12 10.29,15.43 10.29,15.46 X1.3 | 12.66,18.17 Z1.1
D-
  Bottom 0.406: R4.1 14.57,13.28 14.57,11.66 13.74,10.83 Z2.1 12.66,10.8 12.17,10.8 11.32,11.66 11.32,13.89 10.57,14.63 10.57,14.66 X1.2
GATE_CMD  (via drill 0.6)
  Top 0.406: Q1.4 35.3,51.07 v34.29,50.06
  Bottom 0.406: IC7.7 IC7.6 40.07,38.35 41.32,39.61 42.35,39.61 42.69,39.95 42.69,41.66 41.49,42.86 40.63,42.86 39.09,44.41 39.09,45.78 37.72,47.15 37.72,49.55 37.2,50.06 v34.29,50.06
GND  (via drill 0.6)
  Top 0.406: C21.2 14.4,31.03 v15.77,32.23 16.8,31.2 R15.1 | 20.75,26.58 19.55,27.78 18.35,27.78 17.15,28.98 14.41,28.98 C21.2 | U8.35 20,25.83 20.75,26.58 | C21.2 14.22,28.8 | ICSP.6 28.73,3.09 27.09,3.09 26.21,2.21 LED3.C LED4.C | C15.2 v12.69,14.58 9.27,14.58 8.4,13.72 8.4,11.32 C18.2 8.41,10.45 9.77,9.09 9.77,8.82 L2.2 10.19,6.59 v9.94,6.34 | IDC.15 IDC.16 1.03,46.34 1.03,22.97 2.57,21.26 2.91,21.26 4.29,19.89 4.29,19.06 3.93,18.71 3.93,16.8 4.29,16.44 4.29,14.06 3.77,13.54 2.91,13.54 1.71,12.34 1.71,10.15 2.43,9.44 JMP1.2 | C37.2 45.42,42.6 D2.A 46.51,44.64 U4.6 46.51,47.78 46.46,47.83 | IDC.15 5.86,47.85 U3.2 13.53,47.85 14.92,46.46 18.41,46.46 | 18.41,46.46 BAT.1 | 20.75,26.58 20.75,23.32 21.43,22.63 22.29,22.63 22.63,22.29 24.35,22.29 U8.P$1 25.37,21.95 28.46,21.95 29.37,21.03 U8.15 31.95,21.03 v32.92,19.89 33.26,20.23 33.43,20.23 35.15,18.52 38.58,18.52 39.43,19.37 39.43,20.57 39.09,20.92 Y2.2 | C7.1 29.32,42.01 v29.15,42.18 | 18.41,46.46 18.41,46.52 19.2,47.32 19.2,47.66 v19.03,47.83 | U1.P$36 U1.P$37 U1.P$38 U1.P$39 U1.P$40 U1.P$41 U1.P$42 | U1.P$42 U1.P$43 U1.P$44 | U1.P$42 57.44,9.35 v57.44,11.83 57.44,14.23 60.52,17.32 60.52,21.43 59.66,22.29 56.58,22.29 v56.06,21.77 56.06,22.29 55.38,22.97 55.38,25.03 54.86,25.55 51.61,25.55 50.06,24 v50.06,18.52 | 51.61,37.06 U1.P$19 | U8.23 28.69,29.55 v29.83,30.86 | 51.61,37.06 51.61,34.98 v52.29,34.29 | C24.1 | LED5.C 7.2,49.45 IDC.15 | 51.61,37.06 51.61,38.58 52.12,39.09 64.29,39.09 64.64,39.43 64.64,49.72 63.44,51.09 59.15,51.09 57.95,52.29 57.95,53.42 PANEL.1 | U7.2 31.55,47.58 C13.2 | JMP1.2 4.29,8.57
  Top 0.406: 4.29,10.29 JMP1.2
  Top 0.813: C24.1 38.75,42.39 38.74,42.4 C11.1 40.12,44.06
  Bottom 0.406: R16.1 34.98,33.85 C5.2 | U5.7 U5.6 U5.5 31.89,50.98 31.89,52.98 32.58,53.66 39.95,53.66 40.29,53.32 40.29,50.92 | 35.28,48.48 C8.2 | 29.4,43.12 29.32,43.21 29.32,47.32 v29.15,47.49 | 29.4,43.12 31.03,41.49 32.92,41.49 33.6,40.81 33.6,39.65 IC7.4 31.36,39.62 30.69,40.29 28.12,40.29 27.6,40.81 27.6,42.86 28.46,43.72 28.46,44.92 27.6,45.78 25.72,45.78 25.2,45.26 25.2,40.98 26.06,40.12 26.06,37.55 26.92,36.69 26.92,34.29 27.35,33.85 R16.1 | v19.03,47.83 19.47,48.27 C3.2 23.07,48.18 24.69,48.18 24.86,48.35 U5.2 | v29.15,42.18 29.15,42.86 29.4,43.12 | v57.44,11.83 60.27,9 SD1.13 53.7,9 SD1.12 SD1.11 | SD1.6 58.25,18.05 57.26,19.03 57.26,21.26 | 57.26,21.26 57.26,21.6 57.95,22.29 63.84,22.29 SD1.9 | 57.26,21.26 56.75,21.77 v56.06,21.77 56.06,22.29 55.38,22.97 55.38,25.03 54.86,25.55 52.12,25.55 49.64,23.07 C4.1 47.23,22.63 37.03,22.63 36.69,22.29 36.69,21.11 IC1.8 35.83,20.23 32.92,20.23 32.58,20.57 v32.92,19.89 | SD1.10 50.39,18.85 v50.06,18.52 | Z2.2 Z1.2 v12.69,14.58 | P1.- 53.15,33.43 v52.29,34.29 | R16.1 28.63,32.23 v29.83,30.86 | IC3.4 47.32,46.33 47.32,45.26 46.9,44.84 43.28,44.84 42.18,45.95 41.58,45.95 C2.1 41.23,46.04 40.29,46.98 v40.29,49.04 40.29,50.92 | R19.1 16.63,33.09 v15.77,32.23 17.32,32.23 21.43,28.12 26.75,28.12 28.12,29.49 28.63,29.49 v29.83,30.86 | ICSP.6 27.02,1.2 9.6,1.2 8.92,1.89 8.92,5.32 v9.94,6.34 | 28.81,47.48 v29.15,47.49 | 29.48,47.48 v29.15,47.49 | 35.01,48.75 C8.2 | U5.2 U5.3 | U5.7 29.99,48.34 v29.15,47.49 | U5.2 28.3,48.34 v29.15,47.49 | 29.32,30.18 v29.83,30.86 | PANEL.1 42.86,53.49 40.29,50.92 | C8.2 32.06,48.27 U5.7
  pour Bottom (hatched): -2.4,56.24 -2.91,-1.37 66.87,-1.71 67.21,42.69 66.69,43.21 57.09,43.21 56.75,42.86 56.75,40.98 56.24,40.46 56.24,40.29 53.84,37.89 49.03,37.89 48.86,41.32 55.21,48.18 57.26,48.18 57.78,48.69 57.78,56.41 57.26,56.92 48.18,56.92 10.97,56.41 9.94,55.89 9.94,53.32 10.97,52.64 13.03,52.64 14.23,51.44 16.12,51.44 17.49,50.06 17.49,47.49 15.77,45.78 15.77,42.18 14.92,41.32 9.94,41.32 8.57,42.69 8.57,46.12 9.77,47.32 9.77,55.89 9.43,56.24
  pour Top (hatched): 66.87,56.06 52.98,56.24 52.98,55.04 56.75,51.44 62.92,51.44 64.29,49.89 64.29,39.78 63.61,39.09 37.72,39.09 37.2,38.58 37.2,34.29 35.49,32.58 33.43,32.58 32.75,33.26 23.32,33.26 22.29,34.29 22.29,36.52 21.95,36.86 12.34,36.86 11.14,38.06 11.32,40.46 8.92,42.86 8.92,45.61 10.29,46.98 10.29,52.64 11.32,53.66 21.43,53.66 21.95,53.15 25.55,53.15 25.55,54.18 23.49,56.24 -2.06,56.06 -2.06,-1.37 66.87,-1.37
  pour Top: 39.6,42.86 39.6,44.75 39.95,45.09 39.95,49.55 40.98,50.58 41.49,50.58 42.01,51.09 42.86,51.09 43.21,50.75 43.21,50.23 43.72,49.72 48.69,49.72 48.86,49.55 48.86,48.86 47.49,47.49 46.29,47.49 45.61,48.18 44.58,48.18 43.89,47.49 43.89,46.46 43.55,46.12 41.15,46.12 40.98,45.95 40.98,42.86
  pour Top: 31.03,53.49 31.03,54.18 30.52,54.69 27.26,54.69 26.4,53.84 26.4,47.32 27.26,46.46 30.86,46.46 31.03,46.63 30.69,46.98 31.72,47.49 30.86,48.35 27.77,48.35 27.43,48.69 27.43,50.75 27.77,51.09 28.8,51.09 29.32,51.61 29.32,52.64 29.83,53.15 30.69,53.15
  pour Top: 27.26,41.49 27.26,42.35 27.77,42.86 31.2,42.86 31.55,42.52 31.55,40.98 32.06,40.46 32.06,39.6 31.72,39.26 30.69,39.26 30,39.95 30,40.46 29.49,40.98 27.77,40.98
GPIO-4
  Top 0.406: R6.1 40.98,21.6 42.52,23.15 43.64,23.15 U1.P$29
GPIO-6
  Top 0.406: U1.P$27 43.64,27.09 42.69,27.09 41.83,27.95 40.54,27.95 R7.1
HWB
  Top 0.406: R15.2 18.51,28.98 19.03,28.46 20.66,28.46 U8.33
IO0
  Top 0.406: IDC.11 6.82,42.9 9.94,39.78 9.94,37.21 12.52,34.63 17.83,34.63 20.92,31.55 20.92,31.03 22.29,29.66 U8.31
IO1
  Top 0.406: IDC.12 3.19,41.73 3.26,41.66 7.03,41.66 9.26,39.43 9.26,36.69 12.17,33.78 17.49,33.78 20.06,31.2 20.06,30.69 21.49,29.26 U8.32
IO2
  Top 0.406: IDC.13 6.34,45.44 11.32,40.46 11.32,37.89 12.69,36.52 18.35,36.52 22.63,32.23 22.63,31.89 23.83,30.69 23.83,28.49 U8.29
IO3
  Top 0.406: IDC.14 3.26,45.37 3.26,44.75 3.77,44.23 6.52,44.23 10.63,40.12 10.63,37.55 12.69,35.49 18.17,35.49 21.77,31.89 21.77,31.55 23.09,30.23 U8.30
MISO  (via drill 0.6)
  Top 0.406: ICSP.1 33.92,7.06 33.43,7.54 33.43,13.89 30.49,16.83 U8.11 | v58.81,20.23 58.81,17.32 56.06,14.57 51.09,14.57 v49.03,12.52
  Bottom 0.406: SD1.7 59.89,19.15 v58.81,20.23 | ICSP.1 33.78,5.87 33.78,7.2 34.12,7.54 35.15,7.54 36,8.4 39.78,8.4 40.63,9.26 42.18,9.26 46.81,13.89 47.66,13.89 v49.03,12.52
MOSI  (via drill 0.6)
  Top 0.406: U8.10 27.89,15.83 28.63,15.09 v30,15.09 32.4,12.69 32.4,6.69 32.58,6.52 32.58,4.39 ICSP.4
  Bottom 0.406: IC1.5 40.51,16.68 39.26,15.43 34.29,15.43 33.78,14.92 31.2,14.92 v30,15.09
N$1  (via drill 0.6)
  Top 0.406: v60.01,28.29 60.01,30.69 62.41,33.09 63.64,33.09 U1.P$12
  Bottom 0.406: IC1.10 37.97,24.26 38.75,23.49 45.95,23.49 46.81,24.35 49.38,24.35 51.26,26.23 54.69,26.23 55.89,27.43 55.89,28.46 56.75,29.32 58.98,29.32 v60.01,28.29
N$2  (via drill 0.6)
  Top 0.406: LED1.C 18,5.49 v17.32,6.17
  Bottom 0.406: R12.2 29.15,25.55 28.98,25.38 28.98,25.03 26.75,22.8 26.75,14.4 26.57,14.23 26.06,14.23 22.97,11.14 21.77,11.14 21.26,11.66 18.52,11.66 18,11.14 18,6.86 v17.32,6.17
N$3
  pour Bottom: 58.43,55.08 58.43,55.14 58.84,55.54 64.11,55.54 65.15,54.5 65.15,54.44 66.02,53.57 66.02,48.65 65.32,47.95 59.47,47.95 58.55,48.88 58.55,54.9 58.49,54.96
N$4
  Top 0.406: LED2.C 13.54,4.31 R13.2
N$5
  Bottom 0.406: IC7.3 29.8,38.35 R10.1 29.75,37.13 28.98,36.35 28.98,36.1 R16.2
N$6  (via drill 0.6)
  Top 0.406: LED4.A 22.12,5.32 22.63,5.83 24.17,5.83 v24.69,6.34 | v40.46,32.06 R7.2
  Bottom 0.406: v24.69,6.34 24.69,8.06 26.57,9.94 27.43,9.94 28.29,10.8 28.29,22.29 29.66,23.66 31.89,23.66 34.98,26.75 34.98,30.35 35.66,31.03 37.38,31.03 37.72,30.69 38.92,30.69 39.61,31.38 39.78,31.38 v40.46,32.06
N$7
  Bottom 0.406: IC7.1 35.47,35.81 36.18,36.52 36.18,38.75 37.03,39.61 38.76,39.61 IC7.5
N$8  (via drill 0.6)
  Top 0.406: R6.2 40.73,19.03 40.73,16.9 39.43,15.6 39.43,11.14 v38.23,9.94 38.75,10.46 | LED3.A 25.74,4.31 26.75,5.32 26.75,7.2 v26.92,7.37
  Bottom 0.406: v26.92,7.37 27.26,7.72 27.26,8.4 28.98,10.12 33.78,10.12 35.15,11.49 36.69,11.49 v38.23,9.94
N$9  (via drill 0.6)
  Top 0.406: v37.03,16.97 v37.03,13.03
  Bottom 0.406: SD1.2 55.1,13.65 52.81,15.95 48.35,15.95 47.41,16.89 46.38,16.89 45.61,16.12 45.61,14.06 41.66,10.12 40.29,10.12 37.38,13.03 v37.03,13.03 | IC1.6 39.26,21.08 39.26,18.86 37.89,17.49 37.55,17.49 v37.03,16.97
N$10
  pour Top: 43.32,55.37 43.32,51.83 43.78,51.37 44.13,51.37 44.71,50.79 45.34,50.79 45.52,50.97 45.52,52.93 45.98,53.4 50.5,53.34 53.57,50.79 53.39,46.1 53.97,45.52 62.49,45.52 63.47,46.51 63.35,49.58 62.66,50.27 58.78,50.27 58.26,50.79 56.06,50.79 54.26,52.59 54.26,53.05 52,55.31 44.76,55.31 44.65,55.42
N$11
  Bottom 0.406: IC1.2 44.32,19.63 44.92,19.03 48.52,19.03 49.72,20.23 49.72,20.4 50.41,21.09 53.66,21.09 57.78,16.97 64.47,16.97 SD1.5
N$12  (via drill 0.6)
  Top 0.406: v40.98,14.92 v40.98,11.83
  Bottom 0.406: SD1.3 55.03,14.75 52.98,16.8 49.03,16.8 47.83,18 45.78,18 44.58,16.8 44.58,14.75 41.66,11.83 v40.98,11.83 | IC1.4 41.83,21.05 41.83,15.77 v40.98,14.92
N$13
  Top 0.406: R8.2 28.9,49.89 29.15,49.89 29.66,50.41 30,50.41 30.6,51 U7.5
N$14  (via drill 0.6)
  Top 0.406: 63.64,27.09 U1.P$9 63.46,26.92 62.24,26.92 61.21,25.89 58.29,25.89 55.89,28.29 53.32,28.29 v52.81,28.8
  Bottom 0.406: IC1.12 40.51,28.68 41.15,29.32 42.35,29.32 43.72,30.69 50.92,30.69 v52.81,28.8
N$15  (via drill 0.6)
  Top 0.406: U1.P$5 62.32,19.12 61.55,19.89 61.55,23.15 60.69,24 58.64,24 56.06,26.58 52.46,26.58 v50.41,28.63
  Bottom 0.406: IC1.15 44.23,27.34 44.23,28.8 44.75,29.32 49.72,29.32 v50.41,28.63
N$16
  Bottom 0.406: Y1.1 43.36,46.52 IC3.1
N$17
  Bottom 0.406: Y1.2 46.68,49.43 44.75,47.49 44.75,46.4 IC3.2
N$18
  Bottom 0.406: IC3.3 46.07,47.44 46.46,47.83 47.83,47.83 48.35,47.32 48.35,46.56 | 55.04,37.38 57.95,40.29 P1.+$2 | 55.04,37.38 60.52,37.38 61.55,36.35 61.55,26.23 60.52,25.2 57.98,25.2 P1.+$1 | 55.04,37.38 54.69,37.72 51.26,37.72 49.72,39.26 49.72,40.81 48.35,42.18 48.35,46.56 | D5.C 49.18,45.74 48.35,46.56
N$19
  Top 0.406: Q1.1 Q1.2 Q1.3
  pour Top: 42.08,55.48 32.86,55.48 31.89,54.35 31.89,51.26 32.23,50.58 33.26,50.58 34.12,51.44 40.46,51.44 42.16,52.58 42.22,53.1
N$20  (via drill 0.6)
  Top 0.406: LED5.A 6.84,54.35 6.34,54.35 6,54.01 6,50.92 v5.49,50.41
  Bottom 0.406: R20.1 10.12,52.29 8.23,50.41 v5.49,50.41
N$30
  Top 0.406: U3.4 12.77,46.9 14.4,45.26 18.52,45.26 19.03,44.75 19.03,41.88 Q2.4
N$31
  pour Top: 23.66,36.35 29.66,36.35 30.18,36.86 30.18,37.89 30.69,38.4 31.72,38.4 31.89,38.23 31.89,37.38 32.4,36.86 32.4,34.63 31.89,34.12 24.35,34.12 23.49,34.98 23.49,36.18
N$47
  pour Top: 49.03,52.46 50.05,52.46 52.46,50.46 52.46,49.89 51.95,49.38 50.75,49.38 50.41,49.72 50.41,50.06 49.72,50.75 49.21,50.75 48.86,51.09
N$54
  pour Top: 48.52,42.86 48.52,44.58 48.86,44.92 48.86,46.98 50.58,46.98 50.92,48.52 52.46,47.83 52.46,45.09 53.32,44.23 62.24,44.23 63.44,43.03 63.44,41.15 62.75,40.46 54.01,40.81 51.78,42.86
P_LEVEL  (via drill 0.6)
  Top 0.406: U8.28 v24.69,32.23 | v16.46,43.72 v16.46,38.75
  Bottom 0.406: v24.69,32.23 24.69,32.06 19.37,32.06 18.86,32.58 18.86,35.33 17.92,36.27 R19.2 16.46,36.44 v16.46,38.75 | R17.1 v16.46,43.72
RD+  (via drill 0.6)
  Top 0.406: U8.4 23.09,13.66 v22.29,12.86
  Bottom 0.406: v22.29,12.86 21.43,12.86 18.35,15.95 R5.2
RD-  (via drill 0.6)
  Top 0.406: U8.3 22.29,15.09 20.4,13.2 v18.69,13.2
  Bottom 0.406: v18.69,13.2 16.55,13.2 R4.2
RESET  (via drill 0.6)
  Top 0.406: v12.34,20.23 11.51,19.57 10.28,19.57 S2.B2 10.13,19.57 10.13,19.37 5.83,19.37 3.77,21.43 3.77,21.77 R11.1 2.39,24.88 D3.A | v25.2,19.37 30.43,19.37 U8.13 31.32,19.43 32.4,18.35 33.95,18.35 35.32,16.97 35.32,11.14 36,10.46 v36,9.94 36,9.26 37.03,8.23 38.92,8.23 39.43,8.74 v43.72,8.74 | v47.66,26.58 47.66,25.03 46.12,23.49 46.12,12.34 v46.81,11.66
  Bottom 0.406: ICSP.5 28.84,8.6 29.32,9.09 35.15,9.09 v36,9.94 | v12.34,20.23 13.54,20.23 16.12,17.66 24.86,17.66 25.37,18.17 25.37,19.2 v25.2,19.37 | IC1.14 43.05,25.7 43.72,25.03 45.43,25.03 46.29,25.89 46.98,25.89 v47.66,26.58 | v43.72,8.74 43.89,8.74 v46.81,11.66
RXBEE  (via drill 0.6)
  Top 0.406: U8.20 39.43,25.03 v39.61,24.86 | v55.04,30 56.24,30 61.38,35.15 63.63,35.15 U1.P$13
  Bottom 0.406: v55.04,30 54.86,29.83 54.86,27.78 54.18,27.09 50.92,27.09 49.03,25.2 46.63,25.2 45.61,24.17 40.29,24.17 v39.61,24.86
RXLED  (via drill 0.6)
  Top 0.406: U8.8 26.29,14.86 26.92,14.23 27.26,14.23 28.29,13.2 28.29,12 26.92,10.63 26.23,10.63 25.89,10.29 25.89,8.74 25.37,8.23 23.15,8.23 v22.46,7.54 | R13.1 13.45,2.4 11.14,2.4 v10.8,2.74
  Bottom 0.406: v10.8,2.74 11.49,3.43 20.4,3.43 22.46,5.49 v22.46,7.54
S0
  Top 0.406: IDC.3 6.18,32.74 8.23,30.69 8.23,24.86 10.46,22.63 16.12,22.63 16.97,21.77 18.83,21.77 U8.40
S1
  Top 0.406: U8.41 16.69,21.03 15.77,21.95 10.12,21.95 7.37,24.69 7.37,30.52 6.34,31.55 3.94,31.55 3.26,32.23 3.26,32.67 IDC.4
S2
  Top 0.406: IDC.5 6.38,35.28 9.94,31.72 9.94,25.55 11.49,24 16.8,24 17.37,23.43 U8.38
S3
  Top 0.406: U8.39 17.15,22.63 16.46,23.32 10.97,23.32 9.09,25.2 9.09,31.2 6.34,33.95 3.43,33.95 3.26,34.12 3.26,35.21 IDC.6
S4
  Top 0.406: U8.36 17.83,25.03 17.32,25.55 12.17,25.55 11.66,26.06 11.66,32.4 6.86,37.21 6.34,37.21 IDC.7
S5
  Top 0.406: U8.37 17.6,24.23 16.97,24.86 11.66,24.86 10.8,25.72 10.8,32.06 6.34,36.52 3.6,36.52 3.26,36.86 3.26,37.75 IDC.8
SCK  (via drill 0.6)
  Top 0.406: U8.9 27.09,15.6 29.32,13.37 30.35,13.37 30.69,13.03 v30.69,11.83 31.38,11.83 ICSP.3
  Bottom 0.406: IC1.3 43.05,14.59 41.83,13.37 39.09,13.37 37.89,14.57 34.8,14.57 31.89,11.66 30.86,11.66 v30.69,11.83
SCL  (via drill 0.6)
  Top 0.406: v41.15,34.98 38.92,32.75 38.92,27.43 39.26,27.09 41.32,27.09 41.83,26.58 41.83,23.83 40.63,22.63 39.26,22.63 39.09,22.8 38.06,22.8 37.38,23.49 37.32,23.43 U8.18 26.12,23.43 v24.35,25.38 | v49.03,34.12 49.03,33.95 50.58,32.4 51.78,32.4 v52.98,31.2
  Bottom 0.406: IC3.6 46.07,39.48 46.46,39.09 46.46,38.75 46.81,38.41 48.01,38.41 48.35,38.06 48.35,35.49 47.83,34.98 | 47.83,34.98 47.06,34.98 R1.1 | v41.15,34.98 41.83,34.98 45.09,31.72 51.61,31.72 52.12,31.2 v52.98,31.2 | 47.83,34.98 48.18,34.98 v49.03,34.12 | 13.37,28.98 15.43,28.98 15.77,29.32 17.32,29.32 20.75,25.89 24,25.89 24.35,25.55 v24.35,25.38 | 13.37,28.98 11.83,28.98 10.46,30.35 10.46,38.41 9.43,39.43 7.2,39.43 6.86,39.09 3.77,39.09 3.26,39.61 3.26,40.29 IDC.10 | IC4.6 11.44,27.04 13.37,28.98
SDA  (via drill 0.6)
  Top 0.406: 42.01,37.72 v42.69,37.03 41.83,37.89 39.95,37.89 39.26,37.21 39.26,34.46 38.06,33.26 38.06,26.75 38.4,26.4 40.29,26.4 40.98,25.72 40.98,24 40.46,23.49 38.58,23.49 37.83,24.23 U8.19 27.89,24.23 v26.75,25.38 | v7.89,37.89 7.89,39.09 6.69,40.29 5.8,40.29 IDC.9
  Bottom 0.406: v42.69,37.03 43.3,36.43 R9.1 44.92,34.29 46.63,32.58 50.23,32.58 50.75,33.09 50.75,36.86 48.01,39.61 47.49,39.61 47.32,39.78 47.32,40.38 IC3.5 | IDC.9 5.8,40.29 10.46,40.29 11.32,39.26 11.32,30.86 12.17,30 15.09,30 15.43,30.35 17.83,30.35 21.09,27.09 25.03,27.09 v26.75,25.38 | IC4.5 7.57,37.52 v7.89,37.89
SLEEP  (via drill 0.6)
  Top 0.406: U8.25 27.09,29.32 28.29,30.52 28.29,31.89 28.98,32.58 31.2,32.58 32.06,31.72 v32.06,30.86
  Bottom 0.406: IC1.11 39.26,27.27 39.26,28.98 40.46,30.18 41.32,30.18 42.35,31.2 42.35,32.92 41.83,33.43 39.61,33.43 38.06,31.89 35.49,31.89 33.78,30.18 32.92,30.18 v32.06,30.86
TXBEE  (via drill 0.6)
  Top 0.406: U8.21 32.86,25.83 34.98,27.95 34.98,29.49 35.32,29.83 36.18,29.83 v36.52,29.49
  Bottom 0.406: 36.69,27.26 IC1.9 36.7,29.31 v36.52,29.49
TXLED  (via drill 0.6)
  Top 0.406: U8.22 30.49,27.92 v31.2,28.63
  Bottom 0.406: R12.1 29.15,28.12 30,28.98 30.86,28.98 v31.2,28.63
UCAP
  Top 0.406: U8.6 24.69,11.14 24.35,10.8 C12.1
UGND  (via drill 0.6)
  Top 0.406: U8.5 23.89,11.89 22.63,10.63 C12.2 22.47,10.12 15.94,10.12 15.6,9.77 15.6,7.72 14.92,7.03 14.92,6 14.57,5.66 12.17,5.66 10.97,4.46 7.72,4.46 6.69,5.49 v6.69,6.34 7.99,7.64 L2.1 7.9,8.49 JMP1.1
  Bottom 0.406: v6.69,6.34 5.83,6.34 4.97,7.2 4.97,11.59 3.7,12.86 3.7,15.35 4.63,16.27 5.61,16.27 6.37,17.03 8.17,17.03 X1.5 8.21,17.03
VBAT
  Top 0.61: U7.3 32.5,49.11 33.09,48.52 33.09,47.23 C13.1
  pour Top: 15.09,53.15 14.23,53.15 13.54,52.46 13.54,51.78 14.23,51.09 16.29,51.09 17.83,49.55 20.75,49.55 21.77,48.52 21.77,45.78 21.09,45.09 21.09,44.41 21.95,43.55 33.95,43.55 34.46,44.06 34.46,47.66 33.43,47.49 32.58,47.49 32.58,46.12 32.23,45.78 26.75,45.78 25.55,46.98 25.55,50.75 24.69,51.61 21.95,51.61 20.75,52.81 19.72,52.81 18.86,51.95 16.29,51.95
VBAT1  (via drill 0.6)
  Top 0.406: Q2.1 Q2.2 Q2.3 | v23.32,41.66 23.66,41.83 | U8.27 25.49,29.78 v26.57,30.86
  Bottom 0.406: IDC.2 IDC.1 2.37,30.2 1.54,31.03 1.54,40.98 2.23,41.66 12.52,41.66 13.03,42.18 22.8,42.18 v23.32,41.66 | 24.2,42.26 23.74,42.26 v23.32,41.66 | 18.77,49.81 18.86,49.89 24.35,49.89 25.33,50.88 U5.4 | 18.77,49.81 17.49,48.52 17.49,46.98 18.69,45.78 22.38,45.78 C3.1 | R20.2 18.1,50.49 18.77,49.81 | v23.32,41.66 24,42.35 24,45.95 24.17,46.12 | C3.1 23.07,46.37 | U5.1 25.3,47.07 24.35,46.12 24.17,46.12 | 24.17,46.12 23.22,46.12 C3.1 | v26.57,30.86 26.57,33.09 24.52,35.15 24.52,40.46 v23.32,41.66
  pour Top: 18,39.78 18,40.12 18.52,40.63 20.75,40.63 20.92,40.81 20.92,41.83 21.77,42.69 25.72,42.69 26.23,42.18 26.23,40.46 26.4,40.29 28.8,40.29 29.49,39.6 29.49,38.58 29.15,38.23 23.49,38.23 23.15,37.89 18.52,37.89 18.17,38.23
VIN  (via drill 0.6)
  Top 0.406: C37.1 47.15,41.07 47.15,43.38 47.78,44.01 U4.7 47.78,49.43 47.32,49.89 44.41,49.89 43.72,50.58 39.43,50.58 38.58,49.72 38.58,49.04 38.23,48.69 34.98,48.69 34.46,48.18 34.46,43.89 34.12,43.55 28.29,43.55 27.77,44.06 v26.75,44.06 22.29,44.06 v22.46,44.23 22.29,44.23
  Bottom 0.406: R17.2 21.95,43.72 v22.46,44.23 | v26.75,44.06 26.75,39.51 R10.2
  other vias: 50.75,41.32 52.12,40.46
  pour Top: 42.86,44.23 43.03,44.23 43.38,43.89 43.72,43.89 43.89,43.72 43.89,40.98 44.41,40.46 46.29,40.46 46.81,40.98 46.81,41.83 51.44,41.83 52.81,40.81 51.78,39.95 43.38,39.95 41.66,41.66 41.66,43.72 42.01,44.06
  pour Bottom: 64.98,46.98 65.67,46.29 65.67,44.41 65.15,43.89 56.24,43.89 55.55,43.21 55.55,41.32 53.32,38.75 50.06,38.75 49.55,39.26 49.55,40.81 55.38,46.98 57.95,46.98
VTPS  (via drill 0.6)
  other vias: 10.63,44.23 13.89,43.55 15.43,48.86 12.34,50.41 13.89,49.38 12.34,44.23
  pour Top: 13.54,37.38 12.86,37.38 11.83,38.4 11.83,41.15 9.77,43.21 9.77,44.75 10.12,45.09 13.03,45.09 14.06,44.06 14.4,44.06 15.09,43.38 15.09,38.4
  pour Top: 11.49,52.64 11.49,49.21 12,48.69 13.89,48.69 14.92,47.66 16.12,47.66 16.63,48.18 16.63,49.38 15.94,50.06 13.54,50.06 12.69,50.92 12.69,52.12 12,52.81
  pour Bottom: 12.86,51.61 11.49,51.61 10.8,50.92 10.8,46.81 9.6,45.61 9.6,43.89 10.46,43.03 14.06,43.03 14.74,43.72 14.74,46.12 16.63,48.01 16.63,49.55 15.77,50.41 14.23,50.41
VUSB  (via drill 0.6)
  Top 0.406: v26.57,12.52 26.23,12.52 25.49,13.26 U8.7 | C24.2 37.04,39.27 37.38,38.92 37.38,33.78 33.43,29.83 v33.43,28.8
  Top 0.813: 37.08,41.01 C24.2 C11.2
  Bottom 0.406: F2.1 22.12,9.26 24.86,12 26.06,12 v26.57,12.52 26.57,12.69 27.6,13.72 27.6,22.63 29.49,24.52 31.55,24.52 33.43,26.4 v33.43,28.8
  pour Top: 35.49,43.72 35.49,48.01 35.83,48.35 38.75,48.35 39.26,47.83 39.26,46.29 38.06,45.09 38.06,44.41 36.52,42.69
XTAL1
  Top 0.406: U8.17 34.97,22.63 R18.1 36.17,21.94 36.52,21.95 37.86,21.95 Y2.3
XTAL2
  Top 0.406: U8.16 33.03,21.83 34.8,20.06 35.14,20.06 R18.2 35.64,19.92 Y2.1
XUSB
  Bottom 0.406: F2.2 11.83,9.26 10.46,10.63 10.46,12.69 9.32,13.83 8.21,13.83 X1.1

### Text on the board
tPlace: + | + | 1
bPlace: SCK Base Board v1.0 | Designed in Barcelona

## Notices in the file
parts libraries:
SparkFun-PowerIC: Licensing: CC v3.0 Share-Alike You are welcome to use this library for commercial purposes.
